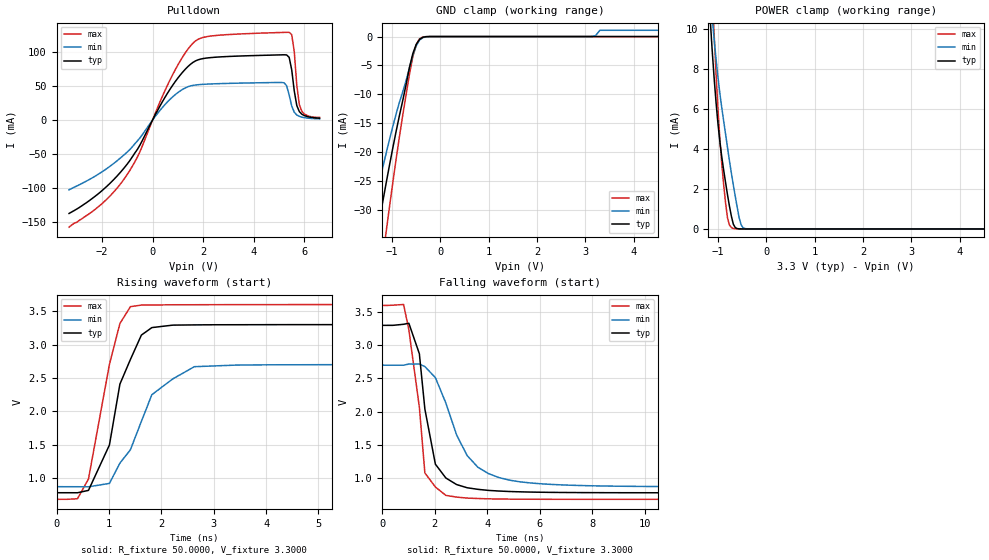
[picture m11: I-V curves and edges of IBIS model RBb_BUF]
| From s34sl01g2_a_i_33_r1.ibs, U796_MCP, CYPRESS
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|   Model RBb_BUF
[Model]  RBb_BUF
Model_type Open_drain
Polarity   Non-Inverting
Enable   Active-High
Vmeas =  1.6500V | Vmeas = Vio*0.5
Cref =   30.0000pF
Rref =   6.2000k
Vref =   3.3000V
C_comp   3.29pF   2.96pF   4.14pF
[Temperature Range]   25.0000   85.0000   -40.0000
[Pullup Reference]   3.3000V   2.7000V   3.6000V
[Pulldown Reference]   0.0V   0.0V   0.0V
[POWER Clamp Reference]   3.3000V   2.7000V   3.6000V
[GND Clamp Reference]   0.0V   0.0V   0.0V
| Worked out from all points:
|   slope of the pulldown table from 0 to 0.495 V, typ, clamps not added: 14.7 ohm
|   GND clamp passes 1 mA (typ) near -0.47 V on its own axis
|   POWER clamp passes 1 mA (typ) near -0.75 V on its own axis
|   rising waveform, R_fixture 50.0000, V_fixture 3.3000: 20-80 % time 536ps typ, 741ps min, 437ps max; typ from 0.779 V to 3.3 V
|   falling waveform, R_fixture 50.0000, V_fixture 3.3000: 20-80 % time 555ps typ, 1.27ns min, 496ps max; typ from 3.3 V to 0.779 V
[Pulldown]
|Voltage   I(typ)   I(min)   I(max)
-3.3V     -137.8mA   -102.9mA   -158mA
-1.1V     -69.56mA   -50.51mA   -85.71mA
900mV     56.9mA     37.59mA    74.42mA
1.8V      88.84mA    52.12mA    119.1mA
5.1V      96.17mA    55.45mA    129.2mA
5.4V      92.37mA    36.76mA    129.4mA
5.5V      73.99mA    20.64mA    126mA
5.6V      43.01mA    11.6mA     101.1mA
5.7V      21.45mA    7.52mA     51.5mA
5.8V      12.51mA    5.49mA     22.8mA
6V        6.58mA     3.52mA     8.9mA
6.6V      2.7mA      1.7mA      4mA
[GND_clamp]
|Voltage   I(typ)   I(min)   I(max)
-3.3V     -993.2mA   -397.9mA   -1.959A
-1.48V    -42.63mA   -33.34mA   -57.88mA
-1.34V    -35.68mA   -28.07mA   -48.21mA
-1.27V    -32.3mA    -25.5mA    -43.51mA
-1.13V    -25.77mA   -20.52mA   -34.37mA
-780mV    -11.16mA   -9.617mA   -13.71mA
-570mV    -2.965mA   -3.308mA   -3.505mA
-500mV    -1.356mA   -1.606mA   -1.413mA
-360mV    -117uA     -187.5uA   -58.29uA
3.14V     756.3pA    21.25uA    371.5pA
3.3V      808.9pA    1.086mA    399pA
6.6V      808.9pA    1.086mA    399pA
[POWER_clamp]
|Voltage   I(typ)   I(min)   I(max)
-3.28V    954.7mA    449.2mA    1.77A
-1.16V    10.56mA    11.89mA    14.41mA
-1.12V    9.036mA    10.68mA    12.1mA
-1.08V    7.645mA    9.57mA     9.906mA
-1V       5.324mA    7.642mA    6.093mA
-960mV    4.398mA    6.817mA    4.554mA
-880mV    2.947mA    5.402mA    2.224mA
-800mV    1.702mA    4.066mA    543.8uA
-680mV    237.8uA    2.197mA    22.81uA
-520mV    1.459uA    215.4uA    122.7nA
-400mV    29.81nA    6.336uA    1.481nA
6.6V      0A         0A         0A
[Ramp]
| variable   typ   min   max
dV/dt_r  1.5058/1.1938n   1.0994/2.2813n   1.7450/0.6751n
dV/dt_f  1.5127/0.6266n   1.0985/1.2033n   1.7520/0.4094n
R_load = 50.0000
[Rising Waveform]
R_fixture= 50.0000
V_fixture= 3.3000
V_fixture_min= 2.7000
V_fixture_max= 3.6000
|time   V(typ)   V(min)   V(max)
0s        778.8mV    869mV      679.7mV
400ps     778.1mV    868.5mV    688.5mV
610ps     814.2mV    867.4mV    984.9mV
1.01ns    1.495V     918.4mV    2.703V
1.21ns    2.407V     1.222V     3.315V
1.41ns    2.775V     1.422V     3.567V
1.62ns    3.142V     1.849V     3.592V
1.82ns    3.254V     2.248V     3.592V
2.63ns    3.294V     2.668V     3.596V
20ns      3.3V       2.7V       3.6V
[Falling Waveform]
R_fixture= 50.0000
V_fixture= 3.3000
V_fixture_min= 2.7000
V_fixture_max= 3.6000
|time   V(typ)   V(min)   V(max)
0s        3.3V       2.7V       3.6V
810ps     3.316V     2.7V       3.614V
1.01ns    3.331V     2.717V     3.231V
1.41ns    2.872V     2.717V     2.066V
1.62ns    2.039V     2.678V     1.077V
2.02ns    1.21V      2.513V     865.6mV
2.42ns    1.001V     2.129V     739mV
3.23ns    854.3mV    1.339V     698.4mV
4.85ns    797.5mV    968.1mV    682.8mV
20ns      778.7mV    868.9mV    679.9mV
